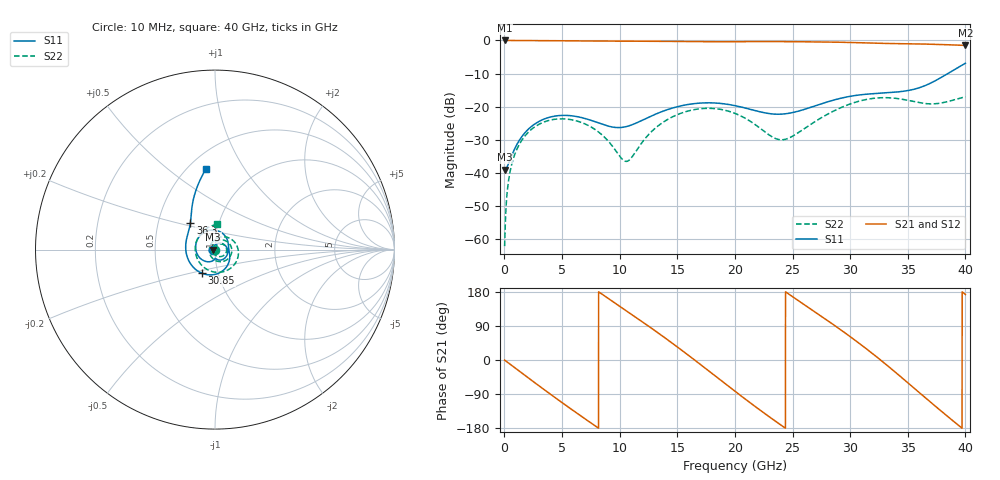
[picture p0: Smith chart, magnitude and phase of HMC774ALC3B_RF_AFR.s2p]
! Analog Devices, Inc.
! 1 Analog Way
! Wilmington, MA 01887
! http://www.analog.com
! Date:  2021-09-17 NN
! Board Name:  EV1HMC774ALC3B Revision A with HMC774ALC3B installed
! File Description:  Automatic Fixture Removal S-Parameters for RF Port connector and board loss de-embedding
! File Generation:  Calibrated Network Analyzer
! Chip Part Number:  HMC774ALC3B
! Chip Description:  MMIC, Double Balanced Mixer
! Chip Frequency:  7 to 34 GHz
! Chip Package:  LCC, 2.9 x 2.9 x 0.8 mm
! RF Port:  HMC774ALC3B removed and end of trace left open
! Note:
!  Analog Devices supplies this data as a sample of measured data at the evaluation board
!  ports for this product.  Your particular data for this product may vary.
!  Analog Devices reserves the right to change this data at anytime.
!  All lines below in this file are as is from the Network Analyzer.
!Agilent Technologies,N5245A,MY52451809,A.10.47.06
!Automatic Fixture Removal (AFR)
!Date: Friday, September 17, 2021 5:43:49 AM
!S2P File: Measurements: S11,S21,S12,S22:
# MHz S  RI  R 50
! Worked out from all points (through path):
!   4000 points, 10 MHz to 40 GHz, reference 50 ohm
!   highest |S21| = 0.00 dB at 10 MHz (marker M1); lowest = -1.5 dB at 40 GHz (marker M2)
!   group delay of S21, straight-line fit = 62.1 ps
!   lowest |S11| = -39.1 dB at 10 MHz (marker M3), VSWR 1.02, Z = 48.9 + j0.0274 ohm
!   |S11| at or under -10 dB: start of sweep to 38.48 GHz
!   |S22| runs from -62.2 to -17.0 dB; largest |S21 - S12| = 1.5e-15
!   S11 on the Smith chart (normalised r, x): 10 MHz: 0.98, +0.00; 30.85 GHz: 0.84, -0.23; 36.3 GHz: 0.73, +0.22; 40 GHz: 0.61, +0.69
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10  -0.0111 0.00028  1 -0.004  1 -0.004  -0.000741 0.000218
520  -0.00808 0.0142  0.9781 -0.2065  0.9781 -0.2065  0.00125 0.0111
1600  0.0144 0.034  0.8006 -0.5949  0.8006 -0.5949  0.0164 0.0283
4070  0.0701 -0.00138  -0.0373 -0.9913  -0.0373 -0.9913  0.0617 0.0128
6680  0.0376 -0.0569  -0.8416 -0.5113  -0.8416 -0.5113  0.0459 -0.0345
8560  0.00785 -0.0529  -0.9689 0.1392  -0.9689 0.1392  0.00876 -0.0349
10550  0.000827 -0.0497  -0.6336 0.7413  -0.6336 0.7413  -0.0146 -0.00255
13340  -0.0422 -0.0677  0.3115 0.9205  0.3115 0.9205  0.0142 0.0492
15140  -0.096 -0.0311  0.8253 0.5014  0.8253 0.5014  0.0598 0.0488
16650  -0.1046 0.0391  0.9573 -0.0586  0.9573 -0.0586  0.0894 0.0174
18160  -0.0568 0.0982  0.7421 -0.6015  0.7421 -0.6015  0.0887 -0.0294
20010  0.0283 0.0992  0.1229 -0.9494  0.1229 -0.9494  0.0426 -0.0663
21600  0.0673 0.0571  -0.4697 -0.839  -0.4697 -0.839  -0.00593 -0.0554
23500  0.0755 0.0137  -0.911 -0.3101  -0.911 -0.3101  -0.0314 -0.00986
26670  0.081 -0.0563  -0.6435 0.7026  -0.6435 0.7026  -0.00141 0.0551
28790  0.0353 -0.1235  0.0317 0.9423  0.0317 0.9423  0.0541 0.0712
30850  -0.0719 -0.132  0.6817 0.6235  0.6817 0.6235  0.1183 0.0282
33340  -0.162 -0.00839  0.8586 -0.2703  0.8586 -0.2703  0.0965 -0.0957
34950  -0.1521 0.0844  0.4652 -0.765  0.4652 -0.765  -0.00551 -0.1248
36300  -0.1372 0.1469  -0.0585 -0.8819  -0.0585 -0.8819  -0.0883 -0.0696
38280  -0.1214 0.2759  -0.7026 -0.5022  -0.7026 -0.5022  -0.0883 0.0766
40000  -0.0507 0.4496  -0.8356 0.1031  -0.8356 0.1031  0.0122 0.1404
